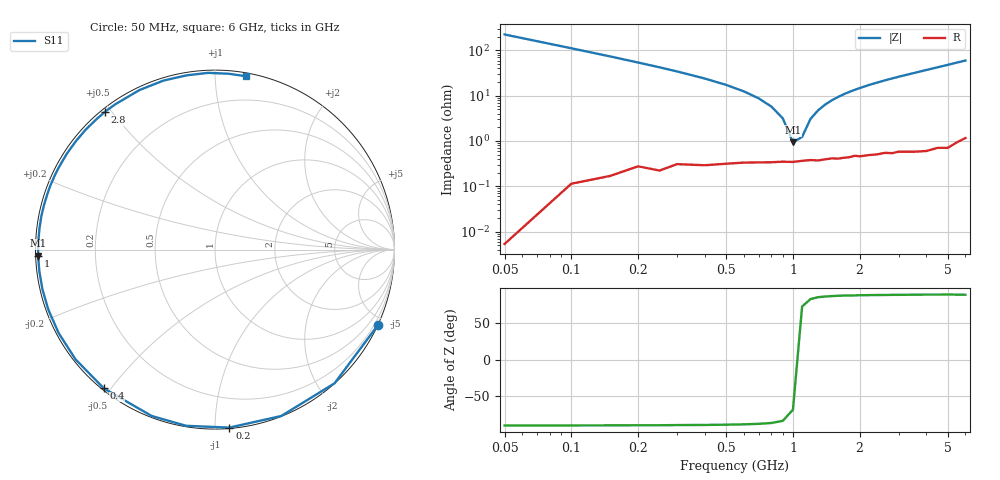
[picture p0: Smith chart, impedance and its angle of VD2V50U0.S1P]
! Infineon Technologies  Discrete & RF Semiconductors
! BBY 55-03
! Si Tuning Diode in SOD323
! VR = 2.5 V
! S-Parameters:  June  1999
# GHz  S  MA  R  50
!  f  S11
! GHz  MAG  ANG
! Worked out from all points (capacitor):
!   34 points, 50 MHz to 6 GHz, reference 50 ohm
!   read as one part to ground: C = 14.1 pF near 50 MHz
!   lowest |Z| = 938 mohm at 1 GHz (marker M1)
!   series resonance near 1.043 GHz, so ESL is about 1.7 nH
!   S11 on the Smith chart (normalised r, x): 50 MHz: 0.00, -4.51; 200 MHz: 0.01, -1.08; 400 MHz: 0.01, -0.48; 1 GHz: 0.01, -0.02; 2.8 GHz: 0.01, +0.48; 6 GHz: 0.02, +1.20
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0.05  1 -25.0
0.1  0.9992 -48.2
0.15  0.9979 -68.3
0.2  0.9949 -85.4
0.25  0.9948 -99.3
0.3  0.9917 -110.9
0.4  0.9906 -128.7
0.5  0.9888 -141.8
0.6  0.9875 -151.9
0.7  0.987 -160.1
0.8  0.9867 -166.9
0.9  0.9862 -172.8
1  0.9863 -178.0
1.2  0.985 173.0
1.3  0.9853 169.1
1.5  0.984 161.9
1.6  0.9843 158.7
1.8  0.9836 152.6
2  0.9833 147.1
2.4  0.9826 137.3
2.8  0.9826 128.6
3  0.982 124.5
3.5  0.9836 115.4
4  0.9846 106.9
4.5  0.9837 99.2
5  0.9854 92.2
5.5  0.9828 85.5
6  0.9811 79.7
